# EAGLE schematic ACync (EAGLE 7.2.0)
DESIGNER: A. Stummer (2015 Feb); GROUP: J. Thywissen Labs; RELEASE_DATE: 2015 Feb; REV: A; TITLE: ACync: AC Line Sync

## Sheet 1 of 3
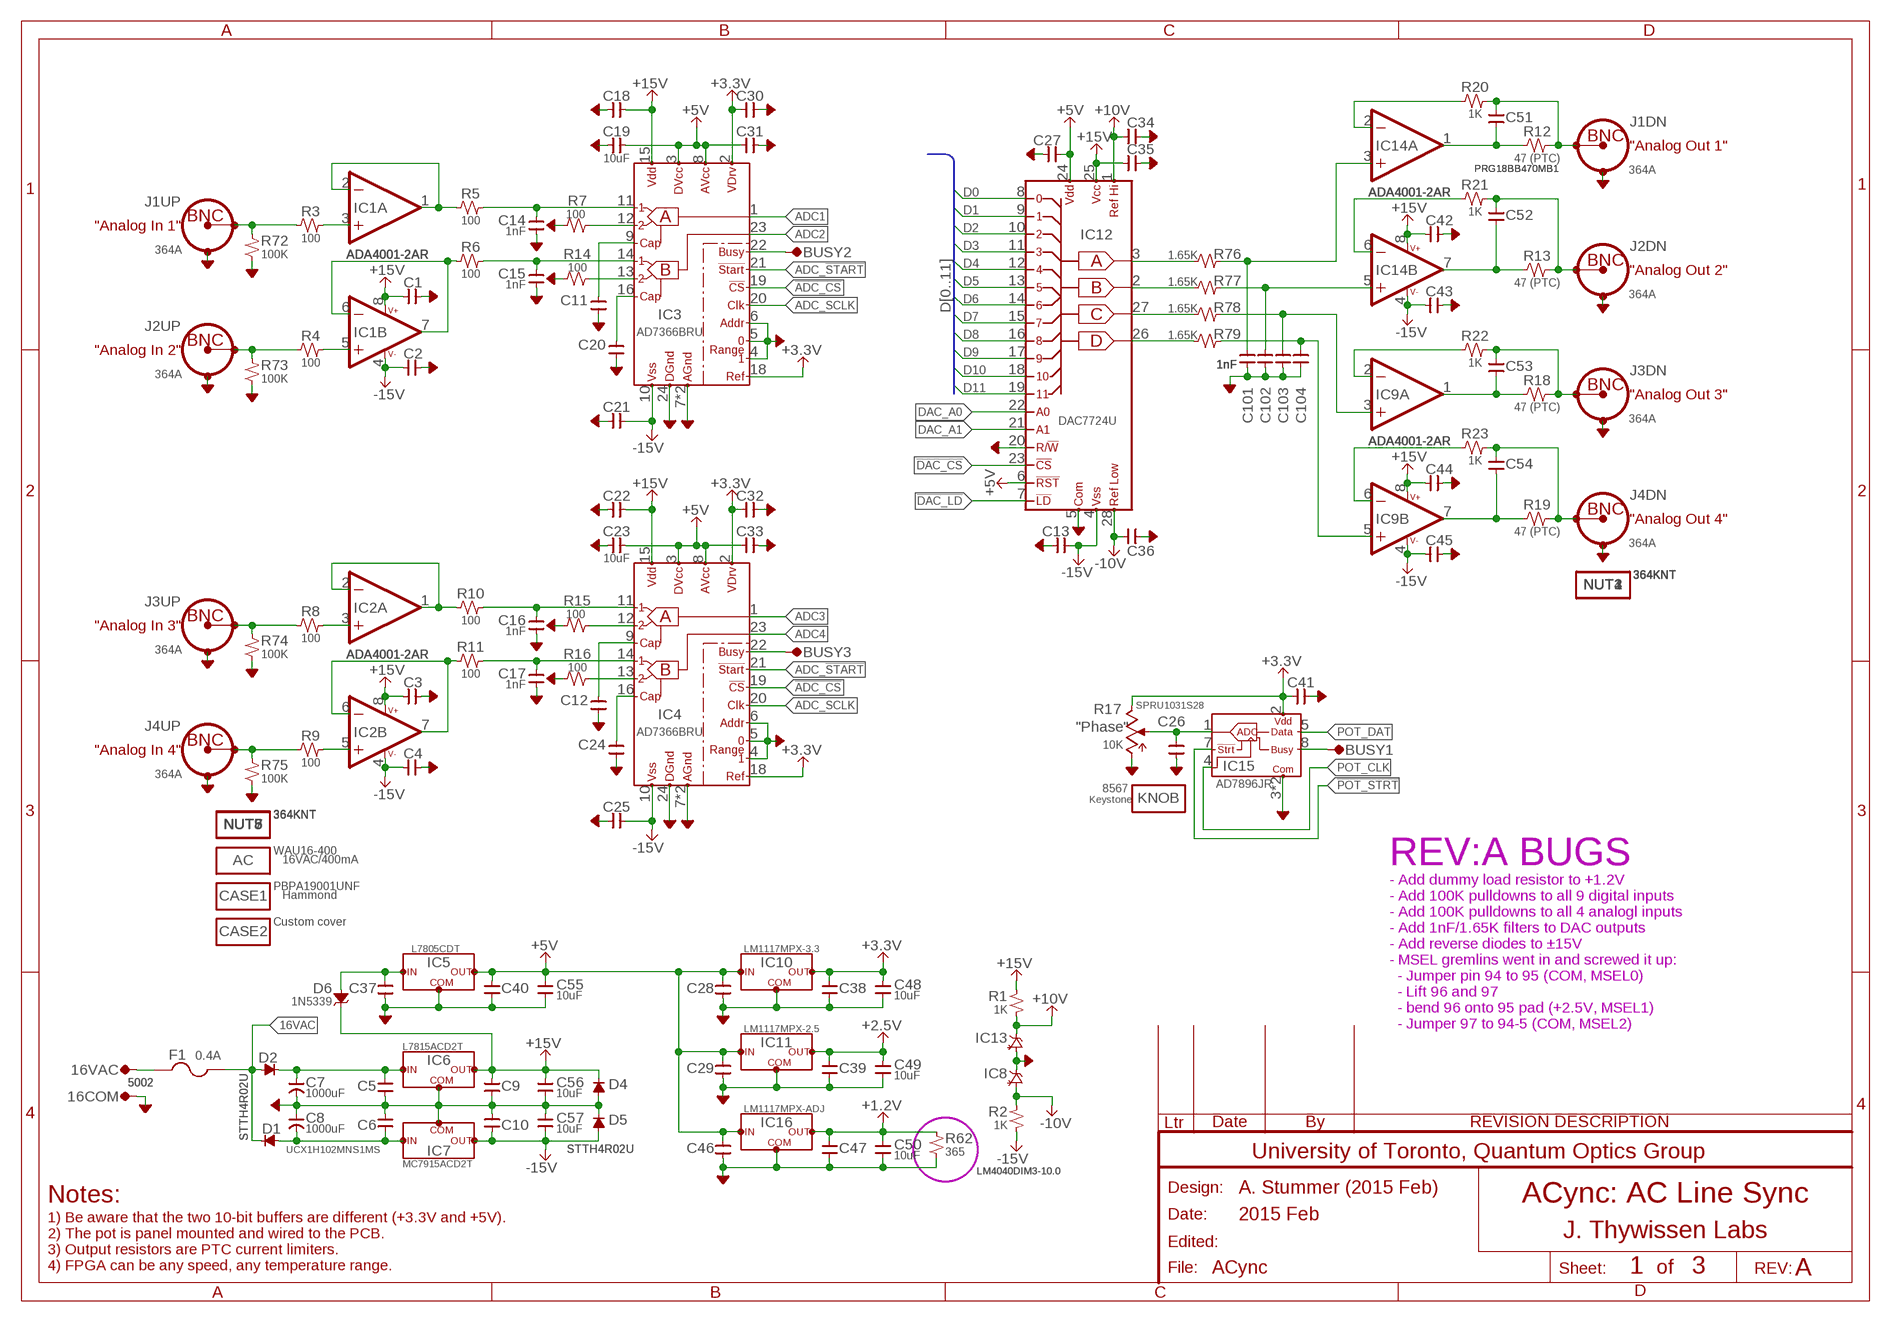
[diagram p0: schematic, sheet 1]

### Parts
16COM  5002  TP-0.042B  [TP-0.042B]
16VAC  5002  TP-0.042B  [TP-0.042B]
AC  WAU16-400  MISC  [MISC]
BUSY1  TP-0.042B  [TP-0.042B]
BUSY2  TP-0.042B  [TP-0.042B]
BUSY3  TP-0.042B  [TP-0.042B]
C1  0.1uF  CAP-H-0805  [2012(0805)]
C2  0.1uF  CAP-H-0805  [2012(0805)]
C3  0.1uF  CAP-H-0805  [2012(0805)]
C4  0.1uF  CAP-H-0805  [2012(0805)]
C5  0.1uF  CAP-V-0805  [2012(0805)]
C6  0.1uF  CAP-V-0805  [2012(0805)]
C7  1000uF  CAP-POL--16MM_SMT  [CAP,POL,16MM,PLASTIC_BASE]
C8  1000uF  CAP-POL--16MM_SMT  [CAP,POL,16MM,PLASTIC_BASE]
C9  0.1uF  CAP-V-0805  [2012(0805)]
C10  0.1uF  CAP-V-0805  [2012(0805)]
C11  0.1uF  CAP-V-0805  [2012(0805)]
C12  0.1uF  CAP-V-0805  [2012(0805)]
C13  0.1uF  CAP-H-0805  [2012(0805)]
C14  1nF  CAP-V-0805  [2012(0805)]
C15  1nF  CAP-V-0805  [2012(0805)]
C16  1nF  CAP-V-0805  [2012(0805)]
C17  1nF  CAP-V-0805  [2012(0805)]
C18  0.1uF  CAP-H-0805  [2012(0805)]
C19  10uF  CAP-H-0805  [2012(0805)]
C20  0.1uF  CAP-V-0805  [2012(0805)]
C21  0.1uF  CAP-H-0805  [2012(0805)]
C22  0.1uF  CAP-H-0805  [2012(0805)]
C23  10uF  CAP-H-0805  [2012(0805)]
C24  0.1uF  CAP-V-0805  [2012(0805)]
C25  0.1uF  CAP-H-0805  [2012(0805)]
C26  0.1uF  CAP-V-0805  [2012(0805)]
C27  0.1uF  CAP-H-0805  [2012(0805)]
C28  0.1uF  CAP-V-0805  [2012(0805)]
C29  0.1uF  CAP-V-0805  [2012(0805)]
C30  0.1uF  CAP-H-0805  [2012(0805)]
C31  0.1uF  CAP-H-0805  [2012(0805)]
C32  0.1uF  CAP-H-0805  [2012(0805)]
C33  0.1uF  CAP-H-0805  [2012(0805)]
C34  0.1uF  CAP-H-0805  [2012(0805)]
C35  0.1uF  CAP-H-0805  [2012(0805)]
C36  0.1uF  CAP-H-0805  [2012(0805)]
C37  0.1uF  CAP-V-0805  [2012(0805)]
C38  0.1uF  CAP-V-0805  [2012(0805)]
C39  0.1uF  CAP-V-0805  [2012(0805)]
C40  0.1uF  CAP-V-0805  [2012(0805)]
C41  0.1uF  CAP-H-0805  [2012(0805)]
C42  0.1uF  CAP-H-0805  [2012(0805)]
C43  0.1uF  CAP-H-0805  [2012(0805)]
C44  0.1uF  CAP-H-0805  [2012(0805)]
C45  0.1uF  CAP-H-0805  [2012(0805)]
C46  0.1uF  CAP-V-0805  [2012(0805)]
C47  0.1uF  CAP-V-0805  [2012(0805)]
C48  10uF  CAP-V-0805  [2012(0805)]
C49  10uF  CAP-V-0805  [2012(0805)]
C50  10uF  CAP-V-0805  [2012(0805)]
C51  0.1uF  CAP-V-0805  [2012(0805)]
C52  0.1uF  CAP-V-0805  [2012(0805)]
C53  0.1uF  CAP-V-0805  [2012(0805)]
C54  0.1uF  CAP-V-0805  [2012(0805)]
C55  10uF  CAP-V-0805  [2012(0805)]
C56  10uF  CAP-V-0805  [2012(0805)]
C57  10uF  CAP-V-0805  [2012(0805)]
C101  1nF  CAP-V-0805  [2012(0805)]
C102  1nF  CAP-V-0805  [2012(0805)]
C103  1nF  CAP-V-0805  [2012(0805)]
C104  1nF  CAP-V-0805  [2012(0805)]
CASE1  PBPA19001UNF  MISC  [MISC]
CASE2  Custom cover  MISC  [MISC]
D1  STTH4R02U  DIODE,GENERIC-SMB  [EIA-B(SMB)]
D2  STTH4R02U  DIODE,GENERIC-SMB  [EIA-B(SMB)]
D4  STTH4R02U  DIODE,GENERIC-SMB  [EIA-B(SMB)]
D5  STTH4R02U  DIODE,GENERIC-SMB  [EIA-B(SMB)]
D6  1N5339  ZENER-THROUGH-0.4"  [PASSIVE_0.4"]
F1  0.4A  FUSE-5X20-4  [FUSE]
IC1  ADA4001-2AR  OPAMP:AD8___(DUAL)-SOIC-8  [SOIC-8]
IC2  ADA4001-2AR  OPAMP:AD8___(DUAL)-SOIC-8  [SOIC-8]
IC3  AD7366BRU  ADC,AD7366/7(12-14-BIT,DUAL,1MSPS,SERIAL)-TSSOP24  [TSSOP-24]
IC4  AD7366BRU  ADC,AD7366/7(12-14-BIT,DUAL,1MSPS,SERIAL)-TSSOP24  [TSSOP-24]
IC5  L7805CDT  REGULATOR:3PIN-D2PAK  [D2PAK]
IC6  L7815ACD2T  REGULATOR:3PIN-D2PAK  [D2PAK]
IC7  MC7915ACD2T  REGULATOR:3PIN-D2PAK(ALT_PINS)  [D2PAK]
IC8  LM4040DIM3-10.0  REFERENCE-3TERMINAL-SHUNT-SOT23  [SOT23]
IC9  ADA4001-2AR  OPAMP:AD8___(DUAL)-SOIC-8  [SOIC-8]
IC10  LM1117MPX-3.3  REGULATOR:LM317(LINEAR,1A,1.25V)EMP  [SOT223]
IC11  LM1117MPX-2.5  REGULATOR:LM317(LINEAR,1A,1.25V)EMP  [SOT223]
IC12  DAC7724U  DAC,QUAD12-BIT,PAR,HV-SOIC28  [SOIC28]
IC13  LM4040DIM3-10.0  REFERENCE-3TERMINAL-SHUNT-SOT23  [SOT23]
IC14  ADA4001-2AR  OPAMP:AD8___(DUAL)-SOIC-8  [SOIC-8]
IC15  AD7896JR  ADC,SERIAL#1-SOIC8  [SOIC-8]
IC16  LM1117MPX-ADJ  REGULATOR:LM317(LINEAR,1A,1.25V)EMP  [SOT223]
J1  364A  CONN:BNC,DUAL-BOMAR_364A  [CONN:BNC,DUAL(BOMAR)]
J2  364A  CONN:BNC,DUAL-BOMAR_364A  [CONN:BNC,DUAL(BOMAR)]
J3  364A  CONN:BNC,DUAL-BOMAR_364A  [CONN:BNC,DUAL(BOMAR)]
J4  364A  CONN:BNC,DUAL-BOMAR_364A  [CONN:BNC,DUAL(BOMAR)]
KNOB  8567  MISC  [MISC]
NUT1  364KNT  MISC  [MISC]
NUT2  364KNT  MISC  [MISC]
NUT3  364KNT  MISC  [MISC]
NUT4  364KNT  MISC  [MISC]
NUT5  364KNT  MISC  [MISC]
NUT6  364KNT  MISC  [MISC]
NUT7  364KNT  MISC  [MISC]
NUT8  364KNT  MISC  [MISC]
R1  1K  R-V-0805  [2012(0805)]
R2  1K  R-V-0805  [2012(0805)]
R3  100  R-H-0805  [2012(0805)]
R4  100  R-H-0805  [2012(0805)]
R5  100  R-H-0805  [2012(0805)]
R6  100  R-H-0805  [2012(0805)]
R7  100  R-H-0805  [2012(0805)]
R8  100  R-H-0805  [2012(0805)]
R9  100  R-H-0805  [2012(0805)]
R10  100  R-H-0805  [2012(0805)]
R11  100  R-H-0805  [2012(0805)]
R12  47 (PTC)  R-H-0603  [1608(0603)]
R13  47 (PTC)  R-H-0603  [1608(0603)]
R14  100  R-H-0805  [2012(0805)]
R15  100  R-H-0805  [2012(0805)]
R16  100  R-H-0805  [2012(0805)]
R17  SPRU1031S28  POT-PRECISION_SPR_RV8  [PRECISION-SPR-RV8(POT)]
R18  47 (PTC)  R-H-0603  [1608(0603)]
R19  47 (PTC)  R-H-0603  [1608(0603)]
R20  1K  R-H-0805  [2012(0805)]
R21  1K  R-H-0805  [2012(0805)]
R22  1K  R-H-0805  [2012(0805)]
R23  1K  R-H-0805  [2012(0805)]
R62  365  R-V-0805  [2012(0805)]
R72  100K  R-V-0805  [2012(0805)]
R73  100K  R-V-0805  [2012(0805)]
R74  100K  R-V-0805  [2012(0805)]
R75  100K  R-V-0805  [2012(0805)]
R76  1.65K  R-H-0805  [2012(0805)]
R77  1.65K  R-H-0805  [2012(0805)]
R78  1.65K  R-H-0805  [2012(0805)]
R79  1.65K  R-H-0805  [2012(0805)]

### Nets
16VAC [Power]: D1.K+(C) D2.A-(A) F1.2A F1.2B(2A) ; also sheet 2
!ADC_CS: IC3.19(!CS) IC4.19(!CS) ; also sheet 2
!DAC_CS: IC12.23(!CS) ; also sheet 2
!DAC_LD: IC12.7(!LDAC) ; also sheet 2
!POT_STRT: IC15.7(!CONVST) ; also sheet 2
+1.2V [Power]: C47.2 C50.2 IC16.2(OUT) R62.2 ; also sheet 2
+2.5V [Power]: C39.2 C49.2 IC11.2(OUT) ; also sheet 2
+3.3V [Power]: C30.1 C32.1 C38.2 C41.1 C48.2 IC3.2(VDRIVE) IC3.18(REFSEL) IC4.2(VDRIVE) IC4.18(REFSEL) IC10.2(OUT) IC15.2(VDD) R17.CW ; also sheet 2
+5V [Power]: C19.2 C23.2 C27.1 C28.2 C29.2 C31.1 C33.1 C40.2 C46.2 C55.2 IC3.3(DVCC) IC3.8(AVCC) IC4.3(DVCC) IC4.8(AVCC) IC5.3(OUT) IC10.3(VI) IC11.3(VI) IC12.6(!RST) IC12.24(VDD) IC16.3(VI) ; also sheet 2
+10V: C34.2 IC12.1(REF-HIGH) IC13.1(A) R1.1
+15V [Power]: C1.2 C3.2 C9.2 C18.2 C22.2 C35.2 C42.2 C44.2 C56.2 D4.K+(C) D6.2(C) IC1.8(PWR:V++) IC2.8(PWR:V++) IC3.15(VDD) IC4.15(VDD) IC6.3(OUT) IC9.8(PWR:V++) IC12.25(VCC) IC14.8(PWR:V++) R1.2
-10V: C36.2 IC8.2(K) IC12.28(REF-LOW) R2.2
-15V [Power]: C2.2 C4.2 C10.2 C13.1 C21.1 C25.1 C43.2 C45.2 C57.1 D5.A-(A) IC1.4(PWR:V-) IC2.4(PWR:V-) IC3.10(VSS) IC4.10(VSS) IC7.3(OUT) IC9.4(PWR:V-) IC12.4(VSS) IC14.4(PWR:V-) R2.1
ADC1: IC3.1(OUTA) ; also sheet 2
ADC2: IC3.23(OUTB) ; also sheet 2
ADC3: IC4.1(OUTA) ; also sheet 2
ADC4: IC4.23(OUTB) ; also sheet 2
ADC_!START: IC3.21(!CNVST) IC4.21(!CNVST) ; also sheet 2
ADC_SCLK: IC3.20(SCLK) IC4.20(SCLK) ; also sheet 2
AGND: 16COM.TP C1.1 C2.1 C3.1 C4.1 C5.1 C6.1 C7.NEG C8.POS C9.1 C10.1 C11.1 C12.1 C13.2 C14.1 C15.1 C16.1 C17.1 C18.1 C19.1 C20.1 C21.2 C22.1 C23.1 C24.1 C25.2 C26.1 C27.2 C28.1 C29.1 C30.2 C31.2 C32.2 C33.2 C34.1 C35.1 C36.1 C37.1 C38.1 C39.1 C40.1 C41.2 C42.1 C43.1 C44.1 C45.1 C46.1 C47.1 C48.1 C49.1 C50.1 C55.1 C56.1 C57.2 C101.1 C102.1 C103.1 C104.1 D4.A-(A) D5.K+(C) IC3.4(RANGE1) IC3.5(RANGE0) IC3.6(ADDR) IC3.7(AGND) IC3.17(AGND) IC3.24(DGND) IC4.4(RANGE1) IC4.5(RANGE0) IC4.6(ADDR) IC4.7(AGND) IC4.17(AGND) IC4.24(DGND) IC5.2(COM) IC5.TAB(COM) IC6.2(COM) IC6.TAB(COM) IC7.1(COM) IC8.1(A) IC10.1(COM) IC11.1(COM) IC12.5(COM) IC12.20(R/!W) IC13.2(K) IC15.3(COM) IC15.6(COM) IC16.1(COM) J1.LWR-COM(DN:SHIELD2) J1.UPR-COM(UP:SHIELD2) J2.LWR-COM(DN:SHIELD2) J2.UPR-COM(UP:SHIELD2) J3.LWR-COM(DN:SHIELD2) J3.UPR-COM(UP:SHIELD2) J4.LWR-COM(DN:SHIELD2) J4.UPR-COM(UP:SHIELD2) R7.1 R14.1 R15.1 R16.1 R17.CCW R62.1 R72.1 R73.1 R74.1 R75.1 ; also sheet 2
D0: IC12.8(D0) ; also sheet 2
D1: IC12.9(D1) ; also sheet 2
D2: IC12.10(D2) ; also sheet 2
D3: IC12.11(D3) ; also sheet 2
D4: IC12.12(D4) ; also sheet 2
D5: IC12.13(D5) ; also sheet 2
D6: IC12.14(D6) ; also sheet 2
D7: IC12.15(D7) ; also sheet 2
D8: IC12.16(D8) ; also sheet 2
D9: IC12.17(D9) ; also sheet 2
D10: IC12.18(D10) ; also sheet 2
D11: IC12.19(D11) ; also sheet 2
DAC_A0: IC12.22(A0) ; also sheet 2
DAC_A1: IC12.21(A1) ; also sheet 2
N$1: C20.2 IC3.16(CAPB)
N$2: C11.2 IC3.9(CAPA)
N$3: C14.2 IC3.11(INA1) R5.2
N$4: C15.2 IC3.14(INB1) R6.2
N$5: IC3.13(INB2) R14.2
N$6: IC3.12(INA2) R7.2
N$7: BUSY2.TP IC3.22(BUSY)
N$8: IC1.1(A:OUT) IC1.2(A:-IN) R5.1
N$9: C51.2 J1.LWR-CTR(DN:CONDUCTOR) R12.2 R20.2
N$10: IC1.6(B:-IN) IC1.7(B:OUT) R6.1
N$11: IC1.3(A:+IN) R3.2
N$12: IC1.5(B:+IN) R4.2
N$13: J2.UPR-CTR(UP:CONDUCTOR) R4.1 R73.2
N$14: J1.UPR-CTR(UP:CONDUCTOR) R3.1 R72.2
N$15: C52.2 J2.LWR-CTR(DN:CONDUCTOR) R13.2 R21.2
N$16: IC14.6(B:-IN) R21.1
N$17: IC9.6(B:-IN) R23.1
N$18: C51.1 IC14.1(A:OUT) R12.1
N$19: C52.1 IC14.7(B:OUT) R13.1
N$20: IC9.2(A:-IN) R22.1
N$21: IC14.2(A:-IN) R20.1
N$22: C53.2 J3.LWR-CTR(DN:CONDUCTOR) R18.2 R22.2
N$23: C54.2 J4.LWR-CTR(DN:CONDUCTOR) R19.2 R23.2
N$24: C53.1 IC9.1(A:OUT) R18.1
N$25: C54.1 IC9.7(B:OUT) R19.1
N$26: C102.2 IC14.5(B:+IN) R77.2
N$27: C101.2 IC14.3(A:+IN) R76.2
N$28: C103.2 IC9.3(A:+IN) R78.2
N$29: C104.2 IC9.5(B:+IN) R79.2
N$30: C24.2 IC4.16(CAPB)
N$31: C12.2 IC4.9(CAPA)
N$32: C16.2 IC4.11(INA1) R10.2
N$33: C17.2 IC4.14(INB1) R11.2
N$34: IC4.13(INB2) R16.2
N$35: IC4.12(INA2) R15.2
N$36: BUSY3.TP IC4.22(BUSY)
N$37: IC2.1(A:OUT) IC2.2(A:-IN) R10.1
N$38: IC2.6(B:-IN) IC2.7(B:OUT) R11.1
N$39: IC2.3(A:+IN) R8.2
N$40: IC2.5(B:+IN) R9.2
N$41: J4.UPR-CTR(UP:CONDUCTOR) R9.1 R75.2
N$42: J3.UPR-CTR(UP:CONDUCTOR) R8.1 R74.2
N$108 [Power-isolated]: 16VAC.TP F1.1A F1.1B(1A)
N$110: BUSY1.TP IC15.8(BUSY)
N$111 [Power]: C6.2 C8.NEG D1.A-(A) IC7.2(VI) IC7.TAB(VI)
N$112 [Power]: C5.2 C7.POS D2.K+(C) IC6.1(VI)
N$113: C26.2 IC15.1(VIN) R17.W
N$121 [Power]: C37.2 D6.1(A) IC5.1(VI)
N$123: IC12.3(QA) R76.1
N$124: IC12.26(QD) R79.1
N$125: IC12.27(QC) R78.1
N$126: IC12.2(QB) R77.1
POT_CLK: IC15.4(SCLK) ; also sheet 2
POT_DAT: IC15.5(SDATA) ; also sheet 2
Unconnected: IC8.3(TRIM) IC13.3(TRIM)

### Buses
D[0..11]

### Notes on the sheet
- "Analog Out 1"
- "Analog In 1"
- "Analog Out 2"
- "Analog In 2"
- "Analog Out 3"
- "Analog Out 4"
- "Analog In 3"
- "Phase"
- 10K
- "Analog In 4"
- 16VAC/400mA | REV:A BUGS
- - Add dummy load resistor to +1.2V
  - Add 100K pulldowns to all 9 digital inputs
  - Add 100K pulldowns to all 4 analogl inputs
  - Add 1nF/1.65K filters to DAC outputs
  - Add reverse diodes to ±15V
  - MSEL gremlins went in and screwed it up:
    - Jumper pin 94 to 95 (COM, MSEL0)
    - Lift 96 and 97
    - bend 96 onto 95 pad (+2.5V, MSEL1)
    - Jumper 97 to 94-5 (COM, MSEL2)
- Hammond
- Notes:
- 1) Be aware that the two 10-bit buffers are different (+3.3V and +5V).
  2) The pot is panel mounted and wired to the PCB.
  3) Output resistors are PTC current limiters.
  4) FPGA can be any speed, any temperature range.

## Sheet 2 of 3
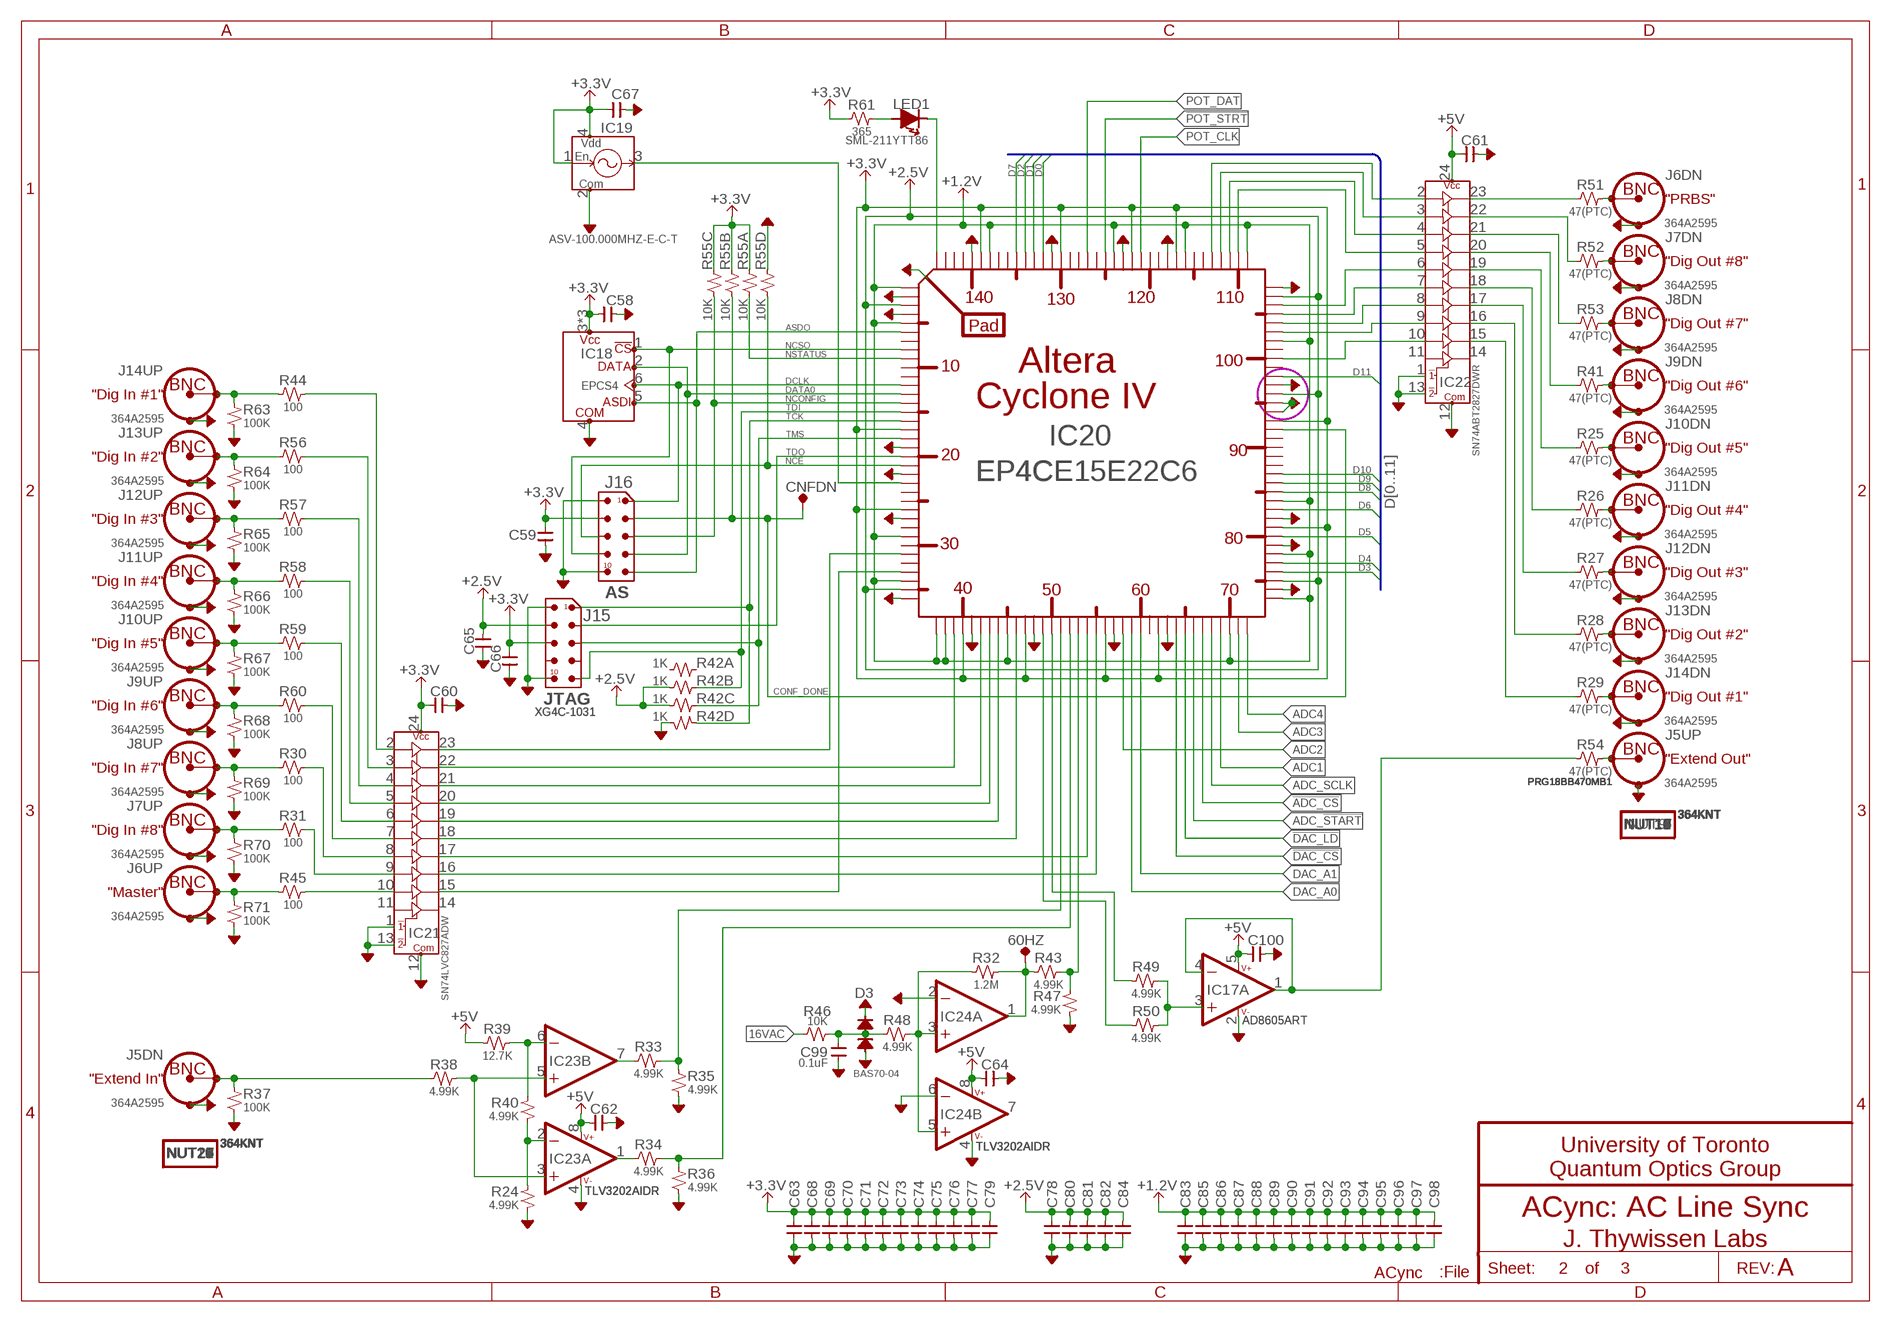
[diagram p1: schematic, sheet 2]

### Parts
60HZ  TP-0.042B  [TP-0.042B]
C58  0.1uF  CAP-H-0805  [2012(0805)]
C59  0.1uF  CAP-V-0805  [2012(0805)]
C60  0.1uF  CAP-H-0805  [2012(0805)]
C61  0.1uF  CAP-H-0805  [2012(0805)]
C62  0.1uF  CAP-H-0805  [2012(0805)]
C63  0.1uF  CAP-V-0402  [1005(0402)]
C64  0.1uF  CAP-H-0805  [2012(0805)]
C65  0.1uF  CAP-V-0805  [2012(0805)]
C66  0.1uF  CAP-V-0805  [2012(0805)]
C67  0.1uF  CAP-H-0805  [2012(0805)]
C68  0.1uF  CAP-V-0402  [1005(0402)]
C69  0.1uF  CAP-V-0402  [1005(0402)]
C70  0.1uF  CAP-V-0402  [1005(0402)]
C71  0.1uF  CAP-V-0402  [1005(0402)]
C72  0.1uF  CAP-V-0402  [1005(0402)]
C73  0.1uF  CAP-V-0402  [1005(0402)]
C74  0.1uF  CAP-V-0402  [1005(0402)]
C75  0.1uF  CAP-V-0402  [1005(0402)]
C76  0.1uF  CAP-V-0402  [1005(0402)]
C77  0.1uF  CAP-V-0402  [1005(0402)]
C78  0.1uF  CAP-V-0402  [1005(0402)]
C79  0.1uF  CAP-V-0402  [1005(0402)]
C80  0.1uF  CAP-V-0402  [1005(0402)]
C81  0.1uF  CAP-V-0402  [1005(0402)]
C82  0.1uF  CAP-V-0402  [1005(0402)]
C83  0.1uF  CAP-V-0402  [1005(0402)]
C84  0.1uF  CAP-V-0402  [1005(0402)]
C85  0.1uF  CAP-V-0402  [1005(0402)]
C86  0.1uF  CAP-V-0402  [1005(0402)]
C87  0.1uF  CAP-V-0402  [1005(0402)]
C88  0.1uF  CAP-V-0402  [1005(0402)]
C89  0.1uF  CAP-V-0402  [1005(0402)]
C90  0.1uF  CAP-V-0402  [1005(0402)]
C91  0.1uF  CAP-V-0402  [1005(0402)]
C92  0.1uF  CAP-V-0402  [1005(0402)]
C93  0.1uF  CAP-V-0402  [1005(0402)]
C94  0.1uF  CAP-V-0402  [1005(0402)]
C95  0.1uF  CAP-V-0402  [1005(0402)]
C96  0.1uF  CAP-V-0402  [1005(0402)]
C97  0.1uF  CAP-V-0402  [1005(0402)]
C98  0.1uF  CAP-V-0402  [1005(0402)]
C99  0.1uF  CAP-V-0805  [2012(0805)]
C100  0.1uF  CAP-H-0805  [2012(0805)]
CNFDN  TP-0.042B  [TP-0.042B]
D3  BAS70-04  DIODE:DUAL(SERIES)-SOT23  [SOT23]
IC17  AD8605ART  OPAMP-SOT23-5  [SOT23-5]
IC18  EPCS4  MEMORY:EPCS1-4(ALTERACONFIG)  [SOIC-8]
IC19  ASV-100.000MHZ-E-C-T  OSCILLATOR:CX750(CITIZEN)-CITIZEN_CSX  [CSX750(CITIZEN_OSC)]
IC20  EP4CE15E22C6  FPGA_EP4C_T144(CYCLONE4)  [EQFP144(TQFP_WITH_GROUND_PAD)]
IC21  SN74LVC827ADW  LOGIC,BUFFER,10-BIT,TRI-SOIC24  [SOIC24]
IC22  SN74ABT2827DWR  LOGIC,BUFFER,10-BIT,TRI-SOIC24  [SOIC24]
IC23  TLV3202AIDR  COMPARATOR:LT1018(4.5NS,DUAL)-SOIC8  [SOIC-8]
IC24  TLV3202AIDR  COMPARATOR:LT1018(4.5NS,DUAL)-SOIC8  [SOIC-8]
J5  364A2595  CONN:BNC,DUAL-BOMAR_364A  [CONN:BNC,DUAL(BOMAR)]
J6  364A2595  CONN:BNC,DUAL-BOMAR_364A  [CONN:BNC,DUAL(BOMAR)]
J7  364A2595  CONN:BNC,DUAL-BOMAR_364A  [CONN:BNC,DUAL(BOMAR)]
J8  364A2595  CONN:BNC,DUAL-BOMAR_364A  [CONN:BNC,DUAL(BOMAR)]
J9  364A2595  CONN:BNC,DUAL-BOMAR_364A  [CONN:BNC,DUAL(BOMAR)]
J10  364A2595  CONN:BNC,DUAL-BOMAR_364A  [CONN:BNC,DUAL(BOMAR)]
J11  364A2595  CONN:BNC,DUAL-BOMAR_364A  [CONN:BNC,DUAL(BOMAR)]
J12  364A2595  CONN:BNC,DUAL-BOMAR_364A  [CONN:BNC,DUAL(BOMAR)]
J13  364A2595  CONN:BNC,DUAL-BOMAR_364A  [CONN:BNC,DUAL(BOMAR)]
J14  364A2595  CONN:BNC,DUAL-BOMAR_364A  [CONN:BNC,DUAL(BOMAR)]
J15  XG4C-1031  CONN:2X5-BLASTER-UNSHROUDED  [CONN,2X5,BLASTER,UNSHROUDED]
J16  XG4C-1031  CONN:2X5-BLASTER-UNSHROUDED  [CONN,2X5,BLASTER,UNSHROUDED]
LED1  SML-211YTT86  LED-0805  [2012(0805)]
NUT9  364KNT  MISC  [MISC]
NUT10  364KNT  MISC  [MISC]
NUT11  364KNT  MISC  [MISC]
NUT12  364KNT  MISC  [MISC]
NUT13  364KNT  MISC  [MISC]
NUT14  364KNT  MISC  [MISC]
NUT15  364KNT  MISC  [MISC]
NUT16  364KNT  MISC  [MISC]
NUT17  364KNT  MISC  [MISC]
NUT18  364KNT  MISC  [MISC]
NUT19  364KNT  MISC  [MISC]
NUT20  364KNT  MISC  [MISC]
NUT21  364KNT  MISC  [MISC]
NUT22  364KNT  MISC  [MISC]
NUT23  364KNT  MISC  [MISC]
NUT24  364KNT  MISC  [MISC]
NUT25  364KNT  MISC  [MISC]
NUT26  364KNT  MISC  [MISC]
NUT27  364KNT  MISC  [MISC]
NUT28  364KNT  MISC  [MISC]
R24  4.99K  R-V-0805  [2012(0805)]
R25  47(PTC)  R-H-0603  [1608(0603)]
R26  47(PTC)  R-H-0603  [1608(0603)]
R27  47(PTC)  R-H-0603  [1608(0603)]
R28  47(PTC)  R-H-0603  [1608(0603)]
R29  47(PTC)  R-H-0603  [1608(0603)]
R30  100  R-H-0805  [2012(0805)]
R31  100  R-H-0805  [2012(0805)]
R32  1.2M  R-H-0805  [2012(0805)]
R33  4.99K  R-H-0805  [2012(0805)]
R34  4.99K  R-H-0805  [2012(0805)]
R35  4.99K  R-V-0805  [2012(0805)]
R36  4.99K  R-V-0805  [2012(0805)]
R37  100K  R-V-0805  [2012(0805)]
R38  4.99K  R-H-0805  [2012(0805)]
R39  12.7K  R-H-0805  [2012(0805)]
R40  4.99K  R-V-0805  [2012(0805)]
R41  47(PTC)  R-H-0603  [1608(0603)]
R42  1K  R-4PAK-0603  [PANASONIC_EXB-V8V(QUAD-R-PACK)]
R43  4.99K  R-H-0805  [2012(0805)]
R44  100  R-H-0805  [2012(0805)]
R45  100  R-H-0805  [2012(0805)]
R46  10K  R-H-0805  [2012(0805)]
R47  4.99K  R-V-0805  [2012(0805)]
R48  4.99K  R-H-0805  [2012(0805)]
R49  4.99K  R-H-0805  [2012(0805)]
R50  4.99K  R-H-0805  [2012(0805)]
R51  47(PTC)  R-H-0603  [1608(0603)]
R52  47(PTC)  R-H-0603  [1608(0603)]
R53  47(PTC)  R-H-0603  [1608(0603)]
R54  47(PTC)  R-H-0603  [1608(0603)]
R55  10K  R-4PAK-0603  [PANASONIC_EXB-V8V(QUAD-R-PACK)]
R56  100  R-H-0805  [2012(0805)]
R57  100  R-H-0805  [2012(0805)]
R58  100  R-H-0805  [2012(0805)]
R59  100  R-H-0805  [2012(0805)]
R60  100  R-H-0805  [2012(0805)]
R61  365  R-H-0805  [2012(0805)]
R63  100K  R-V-0805  [2012(0805)]
R64  100K  R-V-0805  [2012(0805)]
R65  100K  R-V-0805  [2012(0805)]
R66  100K  R-V-0805  [2012(0805)]
R67  100K  R-V-0805  [2012(0805)]
R68  100K  R-V-0805  [2012(0805)]
R69  100K  R-V-0805  [2012(0805)]
R70  100K  R-V-0805  [2012(0805)]
R71  100K  R-V-0805  [2012(0805)]

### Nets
16VAC [Power]: R46.1 ; also sheet 1
!ADC_CS: IC20.67 ; also sheet 1
!DAC_CS: IC20.64 ; also sheet 1
!DAC_LD: IC20.65 ; also sheet 1
!POT_STRT: IC20.125 ; also sheet 1
+1.2V [Power]: C83.2 C85.2 C86.2 C87.2 C88.2 C89.2 C90.2 C91.2 C92.2 C93.2 C94.2 C95.2 C96.2 C97.2 C98.2 IC20.1 IC20.5 IC20.29 IC20.34 IC20.37 IC20.38 IC20.45 IC20.70 IC20.73 IC20.78 IC20.84 IC20.102 IC20.109 IC20.116 IC20.124 IC20.138 ; also sheet 1
+2.5V [Power]: C65.2 C78.2 C80.2 C81.2 C82.2 C84.2 IC20.3 IC20.35 IC20.75 IC20.96 IC20.107 J15.4 R42.2A R42.3A ; also sheet 1
+3.3V [Power]: C58.1 C59.2 C60.1 C63.2 C66.2 C67.1 C68.2 C69.2 C70.2 C71.2 C72.2 C73.2 C74.2 C75.2 C76.2 C77.2 C79.2 IC18.3(VCC3) IC18.7(VCC3) IC18.8(VCC3) IC19.1(EN) IC19.4(VDD) IC20.17 IC20.26 IC20.40 IC20.47 IC20.56 IC20.62 IC20.81 IC20.93 IC20.117 IC20.122 IC20.130 IC20.139 IC21.24(VCC) J15.6 J16.4 R55.1B R55.2B R55.3B R61.1 ; also sheet 1
+5V [Power]: C61.1 C62.2 C64.2 C100.2 IC17.5(B:V++) IC22.24(VCC) IC23.8(V++) IC24.8(V++) R39.1 ; also sheet 1
ADC1: IC20.69 ; also sheet 1
ADC2: IC20.58 ; also sheet 1
ADC3: IC20.71 ; also sheet 1
ADC4: IC20.72 ; also sheet 1
ADC_!START: IC20.66 ; also sheet 1
ADC_SCLK: IC20.68 ; also sheet 1
AGND: C58.2 C59.1 C60.2 C61.2 C62.1 C63.1 C64.1 C65.1 C66.1 C67.2 C68.1 C69.1 C70.1 C71.1 C72.1 C73.1 C74.1 C75.1 C76.1 C77.1 C78.1 C79.1 C80.1 C81.1 C82.1 C83.1 C84.1 C85.1 C86.1 C87.1 C88.1 C89.1 C90.1 C91.1 C92.1 C93.1 C94.1 C95.1 C96.1 C97.1 C98.1 C99.1 C100.1 D3.1(A) D3.2(C) IC17.2(B:V-) IC18.4(COM) IC19.2(COM) IC20.2 IC20.4 IC20.19 IC20.22 IC20.27 IC20.36 IC20.41 IC20.48 IC20.57 IC20.63 IC20.74 IC20.79 IC20.82 IC20.94 IC20.95 IC20.97 IC20.108 IC20.118 IC20.123 IC20.131 IC20.140 IC20.PAD IC21.1(!OE1) IC21.12(COM) IC21.13(!OE2) IC22.1(!OE1) IC22.12(COM) IC22.13(!OE2) IC23.4(V-) IC24.2(A:-IN) IC24.4(V-) IC24.6(B:-IN) J5.LWR-COM(DN:SHIELD2) J5.UPR-COM(UP:SHIELD2) J6.LWR-COM(DN:SHIELD2) J6.UPR-COM(UP:SHIELD2) J7.LWR-COM(DN:SHIELD2) J7.UPR-COM(UP:SHIELD2) J8.LWR-COM(DN:SHIELD2) J8.UPR-COM(UP:SHIELD2) J9.LWR-COM(DN:SHIELD2) J9.UPR-COM(UP:SHIELD2) J10.LWR-COM(DN:SHIELD2) J10.UPR-COM(UP:SHIELD2) J11.LWR-COM(DN:SHIELD2) J11.UPR-COM(UP:SHIELD2) J12.LWR-COM(DN:SHIELD2) J12.UPR-COM(UP:SHIELD2) J13.LWR-COM(DN:SHIELD2) J13.UPR-COM(UP:SHIELD2) J14.LWR-COM(DN:SHIELD2) J14.UPR-COM(UP:SHIELD2) J15.2 J15.10 J16.2 J16.10 R24.1 R35.1 R36.1 R37.1 R42.4B R47.1 R55.4B R63.1 R64.1 R65.1 R66.1 R67.1 R68.1 R69.1 R70.1 R71.1 ; also sheet 1
ASDO: IC18.5(ASDI) IC20.6 J16.9
CONF_DONE: CNFDN.TP IC20.92 J16.3 R55.2A
D0: IC20.132 ; also sheet 1
D1: IC20.133 ; also sheet 1
D2: IC20.134 ; also sheet 1
D3: IC20.76 ; also sheet 1
D4: IC20.77 ; also sheet 1
D5: IC20.80 ; also sheet 1
D6: IC20.83 ; also sheet 1
D7: IC20.135 ; also sheet 1
D8: IC20.85 ; also sheet 1
D9: IC20.86 ; also sheet 1
D10: IC20.87 ; also sheet 1
D11: IC20.98 ; also sheet 1
DAC_A0: IC20.59 ; also sheet 1
DAC_A1: IC20.60 ; also sheet 1
DATA0: IC18.2(DATA) IC20.13 J16.7
DCLK: IC18.6(DCLK) IC20.12 J16.1
N$43: IC20.31 IC21.23(OUT0)
N$44: IC20.39 IC21.22(OUT1)
N$45: IC20.42 IC21.21(OUT2)
N$46: IC20.43 IC21.20(OUT3)
N$47: J6.LWR-CTR(DN:CONDUCTOR) R51.2
N$48: IC22.23(OUT0) R51.1
N$49: J14.LWR-CTR(DN:CONDUCTOR) R29.2
N$50: J13.LWR-CTR(DN:CONDUCTOR) R28.2
N$51: J12.LWR-CTR(DN:CONDUCTOR) R27.2
N$52: J11.LWR-CTR(DN:CONDUCTOR) R26.2
N$53: J10.LWR-CTR(DN:CONDUCTOR) R25.2
N$54: J9.LWR-CTR(DN:CONDUCTOR) R41.2
N$55: J8.LWR-CTR(DN:CONDUCTOR) R53.2
N$56: J14.UPR-CTR(UP:CONDUCTOR) R44.1 R63.2
N$57: IC21.9(IN7) R31.2
N$58: J7.LWR-CTR(DN:CONDUCTOR) R52.2
N$59: IC22.22(OUT1) R52.1
N$60: IC22.21(OUT2) R53.1
N$61: IC22.20(OUT3) R41.1
N$62: IC22.19(OUT4) R25.1
N$63: IC22.18(OUT5) R26.1
N$64: IC22.17(OUT6) R27.1
N$65: IC22.16(OUT7) R28.1
N$66: IC22.15(OUT8) R29.1
N$67: J13.UPR-CTR(UP:CONDUCTOR) R56.1 R64.2
N$68: IC20.100 IC22.10(IN8)
N$69: IC20.103 IC22.9(IN7)
N$70: IC20.104 IC22.8(IN6)
N$71: IC20.105 IC22.7(IN5)
N$72: IC20.106 IC22.6(IN4)
N$73: IC20.110 IC22.5(IN3)
N$74: IC20.111 IC22.4(IN2)
N$75: IC20.44 IC21.19(OUT4)
N$76: IC20.112 IC22.3(IN1)
N$77: IC20.46 IC21.18(OUT5)
N$78: IC20.113 IC22.2(IN0)
N$79: IC20.54 IC21.17(OUT6)
N$80: IC20.55 IC21.16(OUT7)
N$81: IC23.6(B:-IN) R39.2 R40.2
N$82: IC23.2(A:-IN) R24.2 R40.1
N$83: IC21.2(IN0) R44.2
N$84: IC21.3(IN1) R56.2
N$85: IC21.4(IN2) R57.2
N$86: IC21.5(IN3) R58.2
N$87: IC21.6(IN4) R59.2
N$88: IC21.7(IN5) R60.2
N$89: IC21.8(IN6) R30.2
N$90: IC23.3(A:+IN) IC23.5(B:+IN) R38.2
N$91: J5.LWR-CTR(DN:CONDUCTOR) R37.2 R38.1
N$92: IC20.51 R33.2 R35.2
N$93: IC20.52 R34.2 R36.2
N$94: IC20.50 R49.1
N$95: IC20.49 R50.1
N$96: IC17.3(A:+IN) R49.2 R50.2
N$97: J12.UPR-CTR(UP:CONDUCTOR) R57.1 R65.2
N$98: J6.UPR-CTR(UP:CONDUCTOR) R45.1 R71.2
N$99: IC17.1(A:OUT) IC17.4(A:-IN) R54.1
N$100: IC23.1(A:OUT) R34.1
N$101: IC23.7(B:OUT) R33.1
N$102: 60HZ.TP IC24.1(A:OUT) R32.2 R43.1
N$103: IC24.3(A:+IN) IC24.5(B:+IN) R32.1 R48.2
N$104: IC20.53 R43.2 R47.2
N$105: J11.UPR-CTR(UP:CONDUCTOR) R58.1 R66.2
N$106: C99.2 D3.3(MID) R46.2 R48.1
N$107: IC19.3(Q) IC20.23
N$109: J5.UPR-CTR(UP:CONDUCTOR) R54.2
N$114: IC20.33 IC21.15(OUT8)
N$115: J10.UPR-CTR(UP:CONDUCTOR) R59.1 R67.2
N$116: J9.UPR-CTR(UP:CONDUCTOR) R60.1 R68.2
N$117: J8.UPR-CTR(UP:CONDUCTOR) R30.1 R69.2
N$118: J7.UPR-CTR(UP:CONDUCTOR) R31.1 R70.2
N$119: LED1.1(A) R61.2
N$120: IC20.144 LED1.2(C)
N$122: IC21.10(IN8) R45.2
NCE: IC20.21 J16.6 R55.4A
NCONFIG: IC20.14 J16.5 R55.3A
NCSO: IC18.1(NCS) IC20.8 J16.8
NSTATUS: IC20.9 R55.1A
POT_CLK: IC20.121 ; also sheet 1
POT_DAT: IC20.127 ; also sheet 1
TCK: IC20.16 J15.1 R42.4A
TDI: IC20.15 J15.9 R42.2B
TDO: IC20.20 J15.3
TMS: IC20.18 J15.5 R42.3B
Unconnected: IC20.7 IC20.10 IC20.11 IC20.24 IC20.25 IC20.28 IC20.30 IC20.32 IC20.61 IC20.88 IC20.89 IC20.90 IC20.91 IC20.99 IC20.101 IC20.114 IC20.115 IC20.119 IC20.120 IC20.126 IC20.128 IC20.129 IC20.136 IC20.137 IC20.141 IC20.142 IC20.143 IC21.11(IN9) IC21.14(OUT9) IC22.11(IN9) IC22.14(OUT9) IC24.7(B:OUT) J15.7 J15.8 R42.1A R42.1B

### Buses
D[0..11]

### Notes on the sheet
- "PRBS"
- "Dig Out #8"
- "Dig Out #7"
- "Dig Out #6"
- "Dig In #1"
- "Dig Out #5"
- "Dig In #2"
- "Dig Out #4"
- "Dig In #3"
- "Dig Out #3"
- "Dig In #4"
- AS
- "Dig Out #2"
- "Dig In #5"
- JTAG | "Dig Out #1"
- "Dig In #6"
- "Extend Out"
- "Dig In #7"
- "Dig In #8"
- "Master"
- "Extend In"

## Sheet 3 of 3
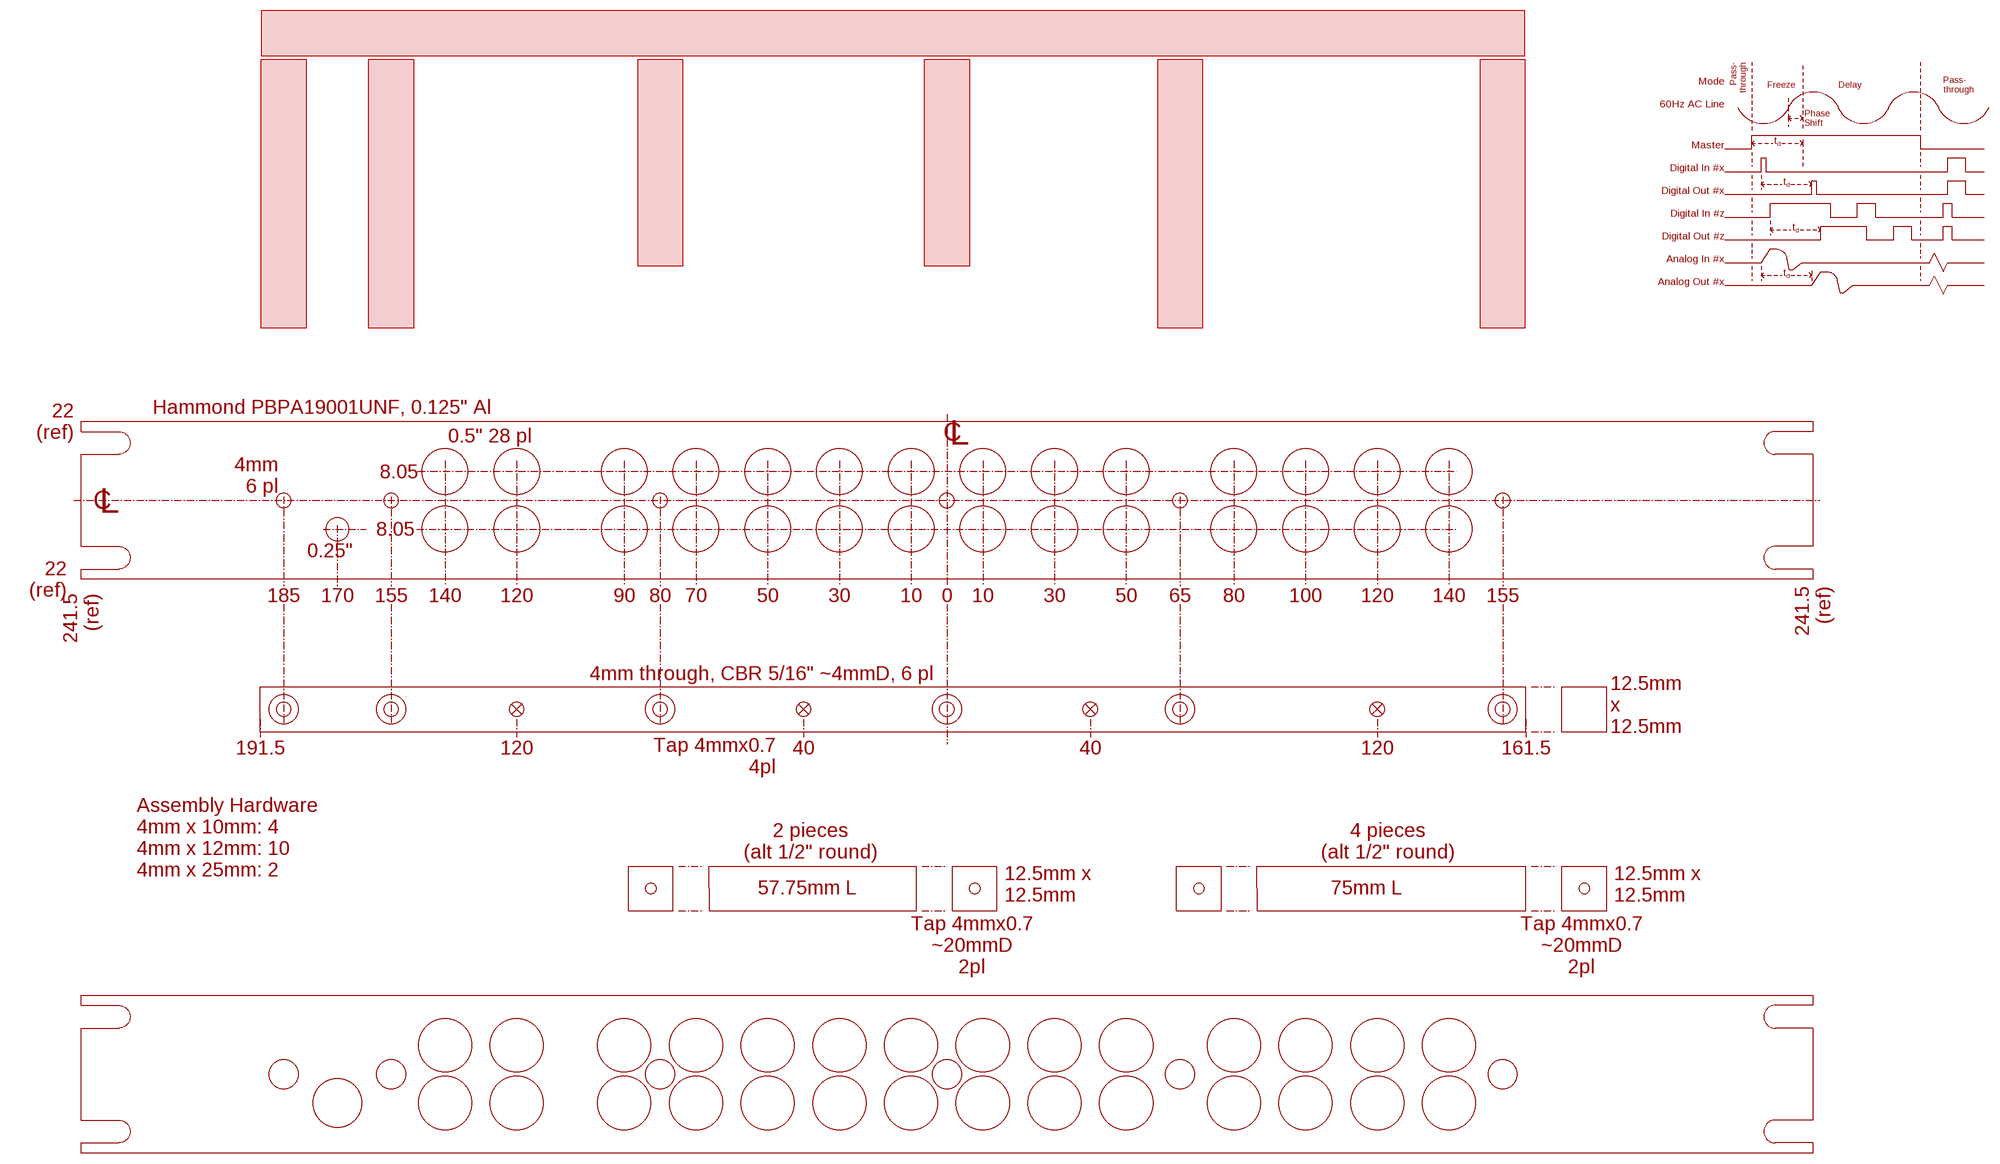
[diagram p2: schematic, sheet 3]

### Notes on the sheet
- Pass-
  through
- Mode | Freeze | Delay
- Pass-
  through
- 60Hz AC Line
- Phase
  Shift
- t | d
- Master
- Digital In #x
- t
- d
- Digital Out #x
- Digital In #z
- t | d
- Digital Out #z
- Analog In #x
- t | d
- Analog Out #x
- Hammond PBPA19001UNF, 0.125" Al
- 22
  (ref)
- 0.5" 28 pl | C | L
- 8.05
- 4mm
  6 pl
- C | L
- 8.05
- 0.25"
- 22
  (ref)
- 241.5
  (ref)
- 185 | 170 | 155 | 140 | 120 | 90 | 80 | 70 | 50 | 30 | 10 | 0 | 10 | 30 | 50 | 65 | 80 | 100 | 120 | 140 | 155
- 241.5
  (ref)
- 4mm through, CBR 5/16" ~4mmD, 6 pl
- 12.5mm
  x
  12.5mm
- Tap 4mmx0.7
  4pl
- 191.5 | 120 | 40 | 40 | 120 | 161.5
- Assembly Hardware
  4mm x 10mm: 4
  4mm x 12mm: 10
  4mm x 25mm: 2
- 2 pieces
  (alt 1/2" round)
- 4 pieces
  (alt 1/2" round)
- 12.5mm x
  12.5mm
- 12.5mm x
  12.5mm
- 57.75mm L | 75mm L
- Tap 4mmx0.7
  ~20mmD
  2pl
- Tap 4mmx0.7
  ~20mmD
  2pl

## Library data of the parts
16COM 16VAC 60HZ BUSY1-BUSY3 CNFDN = QuantumOptics:TP: Testpoint, single pin or single socket, either SMT pad, small hole or loop style TP such as Keystone 5002K (0.042").
AC = QuantumOptics:MISC: Miscellaneous Part, just a placeholder for miscellaeous parts; MFG: CUI
C1-C4 C13 C18 C19 C21-C23 C25 C27 C30-C36 C41-C45 C58 C60-C62 C64 C67 C100 = QuantumOptics:CAP-H-: Cap, SMT and Through-hole, 0402 and up.
C5 C6 C9-C12 C14-C17 C20 C24 C26 C28 C29 C37-C40 C46-C57 C59 C63 C65 C66 C68-C99 C101-C104 = QuantumOptics:CAP-V-: Cap, SMT and Through-hole, 0402 and up.
C7 = QuantumOptics:CAP-POL-: Capacitor, Polarized, SMT 0805 and up, probably tantalum.; PN: UCX1H102MNS1MS
C8 = QuantumOptics:CAP-POL-: Capacitor, Polarized, SMT 0805 and up, probably tantalum.
CASE1 = QuantumOptics:MISC: Miscellaneous Part, just a placeholder for miscellaeous parts; MFG: Hammond
CASE2 NUT1-NUT28 = QuantumOptics:MISC: Miscellaneous Part, just a placeholder for miscellaeous parts
D1 D2 D4 D5 = QuantumOptics:DIODE,GENERIC: Diode, Generic, plain old vanilla diodes.
D3 = QuantumOptics:DIODE:DUAL(SERIES): Dual Diode, series, such as BAS70-04-V in SOT-23
D6 = QuantumOptics:ZENER: Zener
F1 = QuantumOptics:FUSE: Fuse
IC1 IC2 IC9 IC14 = QuantumOptics:OPAMP:AD8___(DUAL): AD8xxx, Analog Devices, dual opamp in SOIC-8 and MSOP-8, various versions available. AD8066, AD8656, etc. e.g. http://www.analog.com/UploadedFiles/Data_Sheets/476080131AD8655_6_a.pdf
IC3 IC4 = QuantumOptics:ADC,AD7366/7(12-14-BIT,DUAL,1MSPS,SERIAL): ADC, dual 12- or 14-bit simultaneous, serial, Analog Devices AD7366/7367.
IC5-IC7 = QuantumOptics:REGULATOR:3PIN: LM1086-xxx, National Semiconductor, LDO, adjustable or fixed. http://cache.national.com/ds/LM/LM1086.pdf
IC8 IC13 = QuantumOptics:REFERENCE-3TERMINAL-SHUNT: Reference, 3 terminal shunt, actually lower power precision supplies, a glorified zener. e.g. http://www.analog.com/en/prod/0,,769_838_ADR525%2C00.html
IC10 IC11 IC16 = QuantumOptics:REGULATOR:LM317(LINEAR,1A,1.25V): LM317, 1.25V bandgap based adjustable regulator. SOT-223 is 1A, D-Pak (TO-252) is 0.5A [sic] http://www.national.com/ds/LM/LM117.pdf
IC12 = QuantumOptics:DAC,QUAD12-BIT,PAR,HV: DAC, quad 12-bit, parallel, uni-bipolar, TI DAC7724, up to ±10V.
IC15 = QuantumOptics:ADC,SERIAL#1: ADC, serial with busy, no ref, such as AD7896.
IC17 = QuantumOptics:OPAMP: Op Amp, generic, pick the right package. e.g. AD8605: SOT-23-5, RRIO, 10MHz, Ib = 1pA, Vio < 65uV, 2.7-5.5V.
IC18 = QuantumOptics:MEMORY:EPCS1-4(ALTERACONFIG): EPCS1 or EPCS4, Altera, FPGA serial configuration device.
IC19 = QuantumOptics:OSCILLATOR:CX750(CITIZEN): CSX750 Oscillators, Citizen, +3.3V or +5V, 1MHZ to 133MHz. http://www.citizencrystal.com/images/pdf/os-csx750f.pdf
IC20 = QuantumOptics:FPGA_EP4C_T144(CYCLONE4): EP4CExxE22xxN, Cyclone IV, Altera FPGA. Pinout is for EP4CE22, can reduce to EP4CE6 for more I/O's and less LE's.
IC21 IC22 = QuantumOptics:LOGIC,BUFFER,10-BIT,TRI: Buffer, 10-bit, tristate, such as TI SN74ABT827/2827.
IC23 IC24 = QuantumOptics:COMPARATOR:LT1018(4.5NS,DUAL): Compatator, dual, Linear Tech, medium fast (4.5nS), single supply to 40V, open drain with weak pullup.
J1-J14 = QuantumOptics:CONN:BNC,DUAL: Dual BNC, vertical throughhole, Bomar, e.g. 364A2595, H=29.3mm, http://media.digikey.com/pdf/Data%20Sheets/Bomar%20PDFs/BNC_Products_Spec.pdf
J15 J16 = QuantumOptics:CONN:2X5-BLASTER: Connector, 2x5 for xBlaster, on 0.1" grid, for Altera FPGA programmer/JTAG connectors. Can use Omron XG4C-1031.
KNOB = QuantumOptics:MISC: Miscellaneous Part, just a placeholder for miscellaeous parts; MFG: Keystone
LED1 = QuantumOptics:LED: LED
R1 R2 R24 R35-R37 R40 R47 R62-R75 = QuantumOptics:R-V-*: Resistor, SMT & Through-Hole, vertical symbol
R3-R11 R14-R16 R20-R23 R30-R34 R38 R39 R43-R46 R48-R50 R56-R61 R76-R79 = QuantumOptics:R-H-*: Resistor, SMT & Through-Hole, horizontal symbol
R12 R13 R18 R19 R25-R29 R41 R51-R54 = QuantumOptics:R-H-*: Resistor, SMT & Through-Hole, horizontal symbol; MFG: Murata; PN: PRG18BB470MB1
R17 = QuantumOptics:POT: Pot, regular or trimpot
R42 R55 = QuantumOptics:R-4PAK: Quad Resistor Pack

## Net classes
0 default: width 0.18 mm, drill 0.508 mm, clearance 0.18 mm
1 Power: width 0.25 mm, drill 0.711 mm, clearance 0.18 mm
2 Power-isolated: width 0.5 mm, drill 0.711 mm, clearance 0.5 mm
